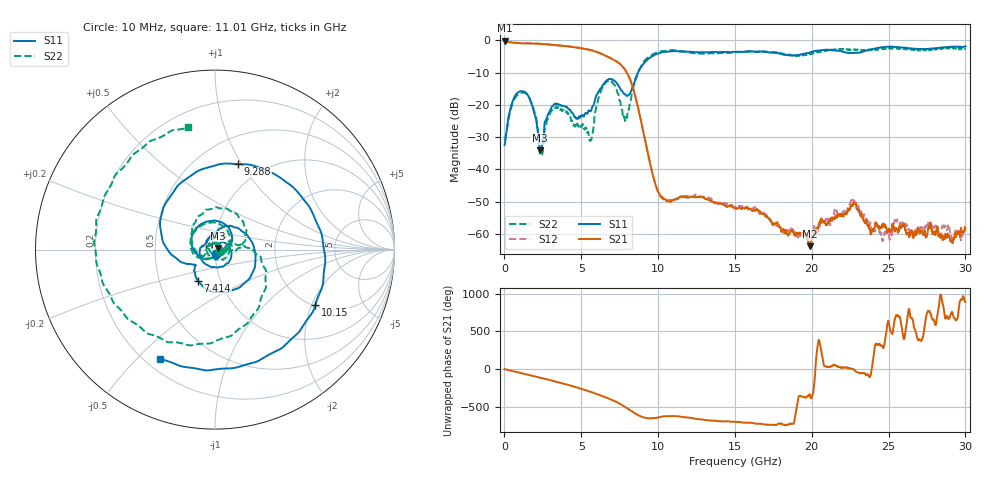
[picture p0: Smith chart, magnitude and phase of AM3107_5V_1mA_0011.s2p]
# Hz S DB R 50.0
!freq dBS11 angS11 dBS21 angS21 dBS12 angS12 dBS22 angS22
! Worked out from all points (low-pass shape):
!   1601 points, 10 MHz to 30 GHz, reference 50 ohm
!   highest |S21| = -0.13 dB at 10 MHz (marker M1); lowest = -63.7 dB at 19.86 GHz (marker M2)
!   |S21| within 3 dB of the highest: start of sweep to 5.658 GHz
!   lowest |S11| = -34.1 dB at 2.315 GHz (marker M3), VSWR 1.04, Z = 51.8 + j0.964 ohm
!   |S11| at or under -10 dB: start of sweep to 8.693 GHz
!   |S22| runs from -35.8 to -2.2 dB; largest |S21 - S12| = 0.011
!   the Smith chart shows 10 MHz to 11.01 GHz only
!   S11 on the Smith chart (normalised r, x): 10 MHz: 1.01, -0.05; 7.414 GHz: 0.78, -0.28; 9.288 GHz: 0.77, +0.96; 10.15 GHz: 2.05, -2.13; 11.01 GHz: 0.26, -0.59
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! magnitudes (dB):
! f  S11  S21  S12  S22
! 10 MHz  -32.5  -0.1  -0.1  -31.0
! 534.8 MHz  -18.8  -0.8  -0.7  -19.4
! 1.153 GHz  -15.8  -1.0  -0.9  -16.3
! 1.847 GHz  -20.8  -1.0  -1.0  -20.4
! 2.315 GHz  -34.1  -1.1  -1.0  -35.1
! 3.309 GHz  -19.6  -1.6  -1.5  -20.7
! 5.015 GHz  -23.3  -2.5  -2.4  -26.7
! 5.652 GHz  -21.6  -3.1  -3.0  -30.7
! 6.608 GHz  -12.7  -4.9  -4.8  -12.8
! 7.414 GHz  -14.0  -7.0  -6.9  -16.7
! 7.864 GHz  -16.8  -9.3  -9.2  -25.0
! 9.288 GHz  -6.1  -34.0  -33.9  -5.6
! 10.02 GHz  -4.1  -47.1  -47.2  -3.7
! 10.15 GHz  -3.9  -48.0  -48.3  -3.5
! 11.01 GHz  -3.3  -49.4  -49.5  -3.1
! 15.01 GHz  -3.6  -52.1  -51.7  -3.7
! 19.86 GHz  -3.9  -63.7  -61.4  -4.2
! 20.01 GHz  -3.6  -60.9  -59.6  -4.2
! 22.67 GHz  -4.0  -51.1  -48.9  -3.1
! 23.87 GHz  -2.8  -59.8  -58.2  -3.0
! 25.01 GHz  -2.0  -58.4  -60.2  -2.6
! 30 GHz  -1.9  -58.2  -57.8  -2.4
